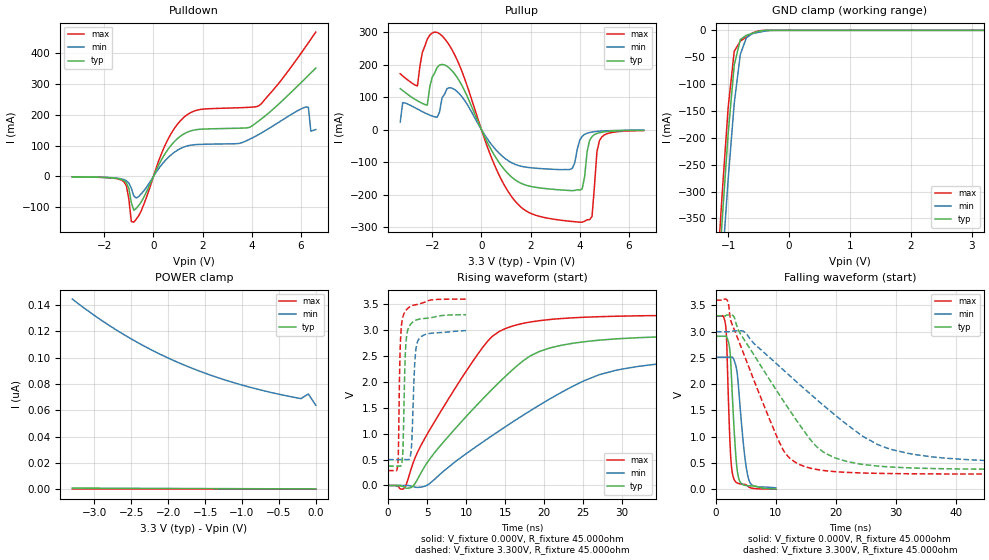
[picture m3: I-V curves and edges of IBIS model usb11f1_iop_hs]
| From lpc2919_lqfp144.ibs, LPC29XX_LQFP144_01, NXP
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| usb11f1
|   Universal Serial Bus Pad
|   Revision 1.1 Specification
|   Programmable Single Ended Core Input
|   Forced Single Ended Low
|   Switchable between
|   - high speed output mode
|   - low speed output mode
|   - low/high speed input mode
| |   Rev 0.20 IBIS Model Design Automation Generation   |
| |   N O N - S I L I C O N   C O R R E L A T E D   |
| |   This IBIS [Model] is pre-Beta tactical support   |
| |  Note: this IBIS [Model] contains clamp curves generated   |
| |   through simulation which should not be relied upon   |
| Pccmos14 hliolib_nlm 4.0
|   0.18 um 3.3V pad library
|   six level metal
|   dual oxide
|   single threshold voltage
|   nominal line mixed supply
|   parasitic extracted netlists
| Process block c14
| High Speed Output Mode
[Model]   usb11f1_iop_hs | of usb11f1
Model_type   I/O
Polarity   Non-Inverting
Enable   Active-Low
|  Reciever Thresholds
Vinl   = 0.8V
Vinh   = 2.0V
| AC Test Load Conditions
Vref   = 0
Cref   = 0
Rref   = 1000000000
Vmeas   = 1.65
| [Process Range]   typical   min   max
| C_comp edge width   400.000ps   400.000ps   400.000ps
| C_comp Tstrobe   40.000fs   40.000fs   40.000fs
C_comp   3.752pF   3.496pF   4.045pF
[Temperature Range]   25   125   -40
[Voltage Range]   3.30V   3.00V   3.60V
[GND Clamp Reference]   0.00V   0.00V   0.00V
[Pulldown Reference]   0.00V   0.00V   0.00V
[POWER Clamp Reference]   3.30V   3.00V   3.60V
[Pullup Reference]   3.30V   3.00V   3.60V
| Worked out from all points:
|   slope of the pulldown table from 0 to 0.495 V, typ, clamps not added: 6.48 ohm
|   slope of the pullup table from 0 to 0.495 V, typ, clamps not added: 6.61 ohm
|   GND clamp passes 1 mA (typ) near -0.46 V on its own axis
|   rising waveform, V_fixture 0.000V, R_fixture 45.000ohm: 20-80 % time 11ns typ, 15.9ns min, 8.17ns max; typ from 0 V to 2.91 V
|   falling waveform, V_fixture 0.000V, R_fixture 45.000ohm: 20-80 % time 847ps typ, 1.21ns min, 606ps max; typ from 2.91 V to 0.006 V
|   rising waveform, V_fixture 3.300V, R_fixture 45.000ohm: 20-80 % time 321ps typ, 402ps min, 285ps max; typ from 0.374 V to 3.3 V
|   falling waveform, V_fixture 3.300V, R_fixture 45.000ohm: 20-80 % time 10.2ns typ, 15.5ns min, 6.95ns max; typ from 3.3 V to 0.374 V
[GND Clamp]
| ref voltage   0.00V   0.00V   0.00V
|   Voltage   I(typ)   I(min)   I(max)
-3.3V     -4.618A    -4.67A     -4.591A
-1.2V     -533.4mA   -616mA     -486.2mA
-1.1V     -356.1mA   -441.1mA   -306.9mA
-1V       -192.1mA   -277.1mA   -143.8mA
-900mV    -64.59mA   -135.6mA   -38.91mA
-800mV    -17.04mA   -44.51mA   -19.95mA
-700mV    -9.237mA   -13.86mA   -12.52mA
-600mV    -5.456mA   -6.064mA   -4.789mA
-500mV    -1.495mA   -3.666mA   -840.2uA
-300mV    -6.625uA   -179.7uA   -408.9nA
3.2V      293.2pA    68.89nA    105.6pA
[Power Clamp]   | Vtable = Vcc - Vpad
| ref voltage   3.30V   3.00V   3.60V
|   Voltage   I(typ)   I(min)   I(max)
-3.3V     1.005nA    144.5nA    354.7pA
-3V       911.2pA    132nA      335.1pA
-2.6V     800.8pA    117.4nA    309pA
-2.3V     727.5pA    108nA      289.6pA
-1.9V     640.7pA    97.15nA    263.8pA
-1.6V     582.9pA    90.25nA    244.5pA
-1.3V     530.6pA    84.3nA     225.3pA
-1V       483pA      79.18nA    206.1pA
-700mV    439.6pA    74.79nA    187pA
-200mV    377.6pA    68.89nA    155pA
-100mV    416.5pA    72.39nA    142.6pA
0V        319.1pA    63.83nA    125.6pA
[Pulldown]
| ref voltage   0.00V   0.00V   0.00V
|   Voltage   I(typ)   I(min)   I(max)
-3.3V     -1.652mA   -1.454mA   -1.796mA
-1.2V     -13.92mA   -10.45mA   -17.73mA
-1.1V     -21.12mA   -14.45mA   -30.61mA
-900mV    -85.23mA   -38.63mA   -146.6mA
-800mV    -110mA     -63.62mA   -148.7mA
500mV     77.03mA    53.28mA    105.7mA
1.1V      130.5mA    90.36mA    180.9mA
4.3V      181mA      136.8mA    229.8mA
6.2V      319.7mA    225.1mA    421.9mA
6.3V      327.6mA    224.1mA    433.3mA
6.4V      335.5mA    146.8mA    444.9mA
6.6V      351.2mA    151.8mA    468.2mA
[Pullup]   | Vtable = Vcc - Vpad
| ref voltage   3.30V   3.00V   3.60V
|   Voltage   I(typ)   I(min)   I(max)
-3.3V     125.8mA    23.2mA     171.5mA
-2.6V     88.3mA     62.98mA    134mA
-2.2V     74.98mA    47.7mA     277.9mA
-1.6V     200.3mA    97.67mA    288.3mA
-1V       161.8mA    117.7mA    216.4mA
900mV     -120mA     -85.3mA    -166.8mA
2.5V      -180.9mA   -120.7mA   -269.8mA
3.7V      -188.1mA   -119.1mA   -283mA
4.1V      -182.9mA   -20.96mA   -285.2mA
4.4V      -34.22mA   -9.287mA   -277.5mA
4.8V      -9.883mA   -5.195mA   -34.66mA
6.6V      -2.365mA   -1.804mA   -3.161mA
[Ramp]
R_load   = 60.000ohm
|   dV/dt(typ)   dV/dt(min)   dV/dt(max)
dV/dt_r   802.872mV/4.105ns   370.430mV/2.890ns   1.330V/4.895ns
dV/dt_f   847.049mV/4.645ns   363.155mV/3.270ns   1.544V/5.270ns
[Rising Waveform]  | cubic spline decimation from 16001 points
V_fixture   = 0.000V
R_fixture   = 45.000ohm
|   Time   V(typ)   V(min)   V(max)
0s        443.9pV    34.48nV    250.2pV
2.065ns   -29.58mV   -1.03uV    -55.15mV
3.17ns    -16.87mV   -18.22mV   416.1mV
5.21ns    482.5mV    23.6mV     1.039V
12.08ns   1.661V     830.7mV    2.652V
16.39ns   2.289V     1.265V     3.095V
21.33ns   2.675V     1.719V     3.211V
26.95ns   2.803V     2.13V      3.257V
32.18ns   2.853V     2.3V       3.275V
80ns      2.912V     2.506V     3.295V
[Falling Waveform]  | cubic spline decimation from 2001 points
V_fixture   = 0.000V
R_fixture   = 45.000ohm
|   Time   V(typ)   V(min)   V(max)
0s        2.914V     2.514V     3.296V
1.64ns    2.92V      2.514V     3.086V
1.765ns   2.904V     2.514V     2.86V
2.38ns    2.57V      2.514V     783.4mV
2.935ns   1.326V     2.481V     213.7mV
3.41ns    505.1mV    2.301V     127.8mV
3.77ns    217.1mV    1.933V     109.5mV
4.66ns    79.74mV    768.8mV    93.98mV
5.445ns   66.7mV     193.7mV    45.74mV
10ns      6.095mV    26.73mV    1.823mV
[Rising Waveform]  | cubic spline decimation from 2001 points
V_fixture   = 3.300V
V_fixture_min = 3.000V
V_fixture_max = 3.600V
R_fixture   = 45.000ohm
|   Time   V(typ)   V(min)   V(max)
0s        373.7mV    499.4mV    287.7mV
1.245ns   373.7mV    499.4mV    398.8mV
1.58ns    374.4mV    499.5mV    2.748V
1.88ns    599.6mV    499.5mV    3.241V
2.075ns   1.793V     499.5mV    3.326V
2.365ns   2.864V     499.5mV    3.393V
2.965ns   3.125V     677.1mV    3.464V
3.435ns   3.18V      2.395V     3.485V
3.815ns   3.203V     2.788V     3.498V
10ns      3.296V     2.989V     3.598V
[Falling Waveform]  | cubic spline decimation from 16001 points
V_fixture   = 3.300V
V_fixture_min = 3.000V
V_fixture_max = 3.600V
R_fixture   = 45.000ohm
|   Time   V(typ)   V(min)   V(max)
0s        3.3V       3V         3.6V
1.905ns   3.316V     3V         3.592V
2.51ns    3.319V     3V         3.198V
5.015ns   2.793V     2.974V     2.463V
11.14ns   1.702V     2.283V     764.9mV
14.69ns   1.108V     1.918V     436.9mV
20.36ns   578.2mV    1.367V     331.2mV
27ns      441.4mV    850.1mV    302.8mV
32.03ns   408.2mV    684.4mV    295.3mV
80ns      374.5mV    503.6mV    287.9mV
